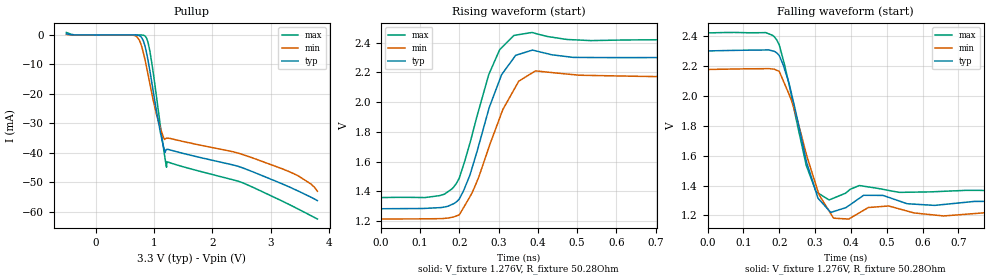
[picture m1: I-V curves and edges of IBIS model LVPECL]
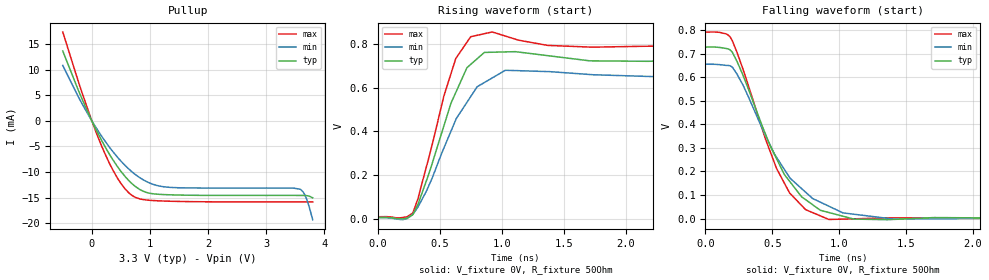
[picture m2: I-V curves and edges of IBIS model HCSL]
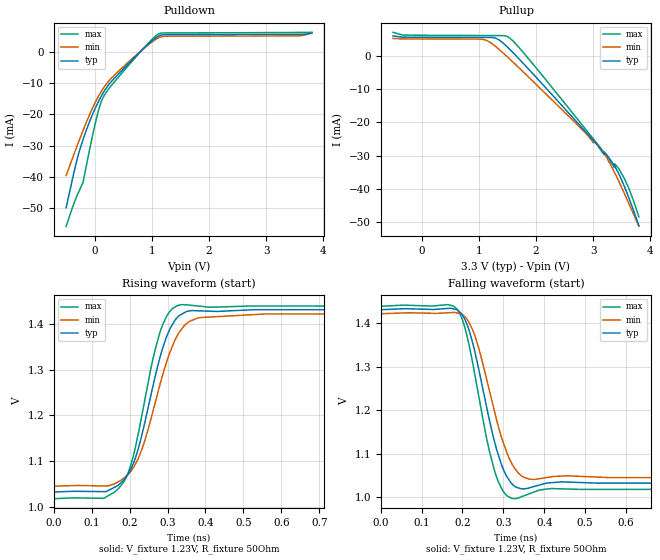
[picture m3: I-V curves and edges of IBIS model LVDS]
|Texas Instruments Incorporated
| Marketing part#   Digital Voltage Range   Package-type   #pins
|   LMK61E2   3.15V - 3.465V
[IBIS Ver]   4.1
[File name]   lmk61e2.ibs
[File Rev]   1.0
[Date]   08/25/2015
[Source]
| Texas Instruments Incorporated.
| 12500 TI Blvd
| Dallas, TX -75243
[Notes]   Revision History:
| Rev 1.0: 08/25/2015
| - Initial version of the model
| - Model generated from simulations in TISPICE
| - C_comp although listed in numerical order of value are
|   obtained from varying PVT conditions. For PVT conditions for
|   each specific value refer the buffer description under
|   respective [Model]. IBIS model user is responsible for using
|   appropriate C_comp to simulate for Signal Integrity.
| - Warnings regarding combined Non-monotonicity of various models have been
|   reviewd and considered minor and can be ignored.
| - Model DRV has sub modles, LVPECL, HCSL, LVDS, depending on the
|   driver mode. User should be able to select a desired driver under
|   [Model Selector].
[Disclaimer]
| This model is designed as an aid for customers of Texas Instruments.
| TI and its licensors and suppliers make no warranties, either expressed
| or implied, with respect to this  model, including the warranties of
| merchantability or fitness for a particular purpose. The model is
| provided solely on an "as is" basis. The entire risk as to its quality
| and performance is with the customer.
[Copyright]
 (C) Copyright 2015 Texas Instruments Incorporated.All rights reserved.
|   Device
[Component] LMK61E2
[Manufacturer]   TI
[Package]
|   typ   min   max
R_pkg   0   0   0
L_pkg   0   0   0
C_pkg   0   0   0
[Pin]  signal_name model_name   R_pin   L_pin   C_pin
1   OE   NC   0   0   0
2   ADD   NC   0   0   0
3   GND   GND   0   0   0
4   OUTP   DRV  0   0   0
5   OUTN   DRV   0   0   0
6   VCC   POWER   0   0   0
7   SDA   NC   0   0   0
8   SCL   NC   0   0   0
[Diff Pin]  inv_pin  vdiff  tdelay_typ tdelay_min tdelay_max
4   5   NA   NA   NA   NA
|   Model Selectors
[Model Selector]  DRV
LVPECL  driver in lvpecl mode
HCSL  driver in hcsl mode
LVDS  driver in lvds mode
| Models and submodels in the file (3): LVPECL (Open_source), HCSL (Open_source), LVDS (Output)
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|   Model
[Model]   LVPECL
Model_type   Open_source
Polarity   Non-Inverting
Vmeas = 1.6
Vref = 1.276
Cref = 1pF
Rref = 50
|   typ   min   max
C_comp   0.215pF   0.202pF   0.225pF
[Voltage Range]   3.3   3.135   3.465
[Temperature Range]   27   85   -40
[Pullup Reference]   3.3   3.135   3.465
[Pulldown Reference]   0   0   0
[Power Clamp Reference]   3.3   3.135   3.465
[GND Clamp Reference]   0   0   0
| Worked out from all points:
|   falling waveform, V_fixture 1.276V, R_fixture 50.28Ohm: 20-80 % time 59.3ps typ, 70.2ps min, 57.1ps max; typ from 2.3 V to 1.29 V
|   rising waveform, V_fixture 1.276V, R_fixture 50.28Ohm: 20-80 % time 72.3ps typ, 83.7ps min, 68.7ps max; typ from 1.28 V to 2.31 V
[Pullup]
|   Voltage   I(typ)   I(min)   I(max)
-500mV    388.3uA    158.6uA    847.9uA
656.7mV   -6.836uA   -136.4uA   -40.3nA
759.9mV   -323uA     -2.236mA   -5.545uA
863.1mV   -5.164mA   -9.896mA   -731.8uA
936.2mV   -12.86mA   -17.1mA    -6.174mA
1.117V    -33.67mA   -32.01mA   -31.83mA
1.19V     -39.75mA   -35.29mA   -41.82mA
1.216V    -38.82mA   -35mA      -44.83mA
1.233V    -38.78mA   -34.98mA   -43.02mA
2.446V    -44.54mA   -40.07mA   -49.58mA
3.465V    -52.84mA   -47.68mA   -58.94mA
3.8V      -56.16mA   -52.97mA   -62.4mA
[Ramp]
R_load = 50.28
|   typ   min   max
dV/dt_r   0.613874/7.22802e-11   0.581205/8.37044e-11   0.635139/6.87025e-11
dV/dt_f   0.605179/9.77e-11   0.573672/7.01775e-11   0.633996/5.71456e-11
[Falling Waveform]
V_fixture = 1.276V
V_fixture_min = 1.212V
V_fixture_max = 1.34V
R_fixture = 50.28Ohm
C_fixture = 0F
|   Time   V(typ)   V(min)   V(max)
0s        2.298V     2.174V     2.418V
162.1ps   2.304V     2.179V     2.42V
200ps     2.267V     2.162V     2.338V
227.2ps   2.083V     2.009V     2.076V
275ps     1.569V     1.615V     1.537V
307.8ps   1.316V     1.362V     1.35V
339.1ps   1.233V     1.23V      1.304V
435.5ps   1.335V     1.235V     1.395V
633.7ps   1.267V     1.203V     1.359V
2ns       1.289V     1.218V     1.361V
[Rising Waveform]
V_fixture = 1.276V
V_fixture_min = 1.212V
V_fixture_max = 1.34V
R_fixture = 50.28Ohm
C_fixture = 0F
|   Time   V(typ)   V(min)   V(max)
0s        1.284V     1.215V     1.359V
149.5ps   1.291V     1.218V     1.372V
200ps     1.349V     1.243V     1.49V
227.2ps   1.511V     1.365V     1.725V
275ps     1.952V     1.694V     2.184V
307.8ps   2.185V     1.929V     2.365V
339.1ps   2.298V     2.083V     2.448V
393.9ps   2.345V     2.21V      2.461V
534.8ps   2.299V     2.179V     2.413V
2ns       2.307V     2.184V     2.418V
|   Model
[Model]   HCSL
Model_type   Open_source
Polarity   Non-Inverting
Vmeas = 0.35
Vref = 0
Cref = 1pF
Rref = 50
|   typ   min   max
C_comp   0.215pF   0.202pF   0.225pF
[Voltage Range]   3.3   3.135   3.465
[Temperature Range]   27   85   -40
[Pullup Reference]   3.3   3.135   3.465
[Pulldown Reference]   0   0   0
[Power Clamp Reference]   3.3   3.135   3.465
[GND Clamp Reference]   0   0   0
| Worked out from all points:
|   slope of the pullup table from 0 to 0.495 V, typ, clamps not added: 50.6 ohm
|   falling waveform, V_fixture 0V, R_fixture 50Ohm: 20-80 % time 347ps typ, 395ps min, 301ps max; typ from 0.728 V to 0 V
|   rising waveform, V_fixture 0V, R_fixture 50Ohm: 20-80 % time 256ps typ, 312ps min, 216ps max; typ from 0.005 V to 0.727 V
[Pullup]
|   Voltage   I(typ)   I(min)   I(max)
-500mV    13.64mA    10.81mA    17.35mA
-164.6mV  4.159mA    3.265mA    5.36mA
11.7mV    -280.2uA   -219.3uA   -362.8uA
175.1mV   -3.963mA   -3.111mA   -5.088mA
441.7mV   -8.953mA   -7.106mA   -11.2mA
575mV     -10.91mA   -8.74mA    -13.33mA
695.4mV   -12.31mA   -9.994mA   -14.59mA
936.2mV   -13.96mA   -11.83mA   -15.45mA
1.297V    -14.42mA   -12.95mA   -15.68mA
3.585V    -14.56mA   -13.35mA   -15.82mA
3.684V    -14.59mA   -14.95mA   -15.82mA
3.8V      -15.04mA   -19.3mA    -15.83mA
[Ramp]
R_load = 50
|   typ   min   max
dV/dt_r   0.433319/2.55754e-10   0.391319/3.11773e-10   0.469787/2.15724e-10
dV/dt_f   0.436287/3.47027e-10   0.392611/3.95051e-10   0.474509/3.01064e-10
[Falling Waveform]
V_fixture = 0V
V_fixture_min = 0V
V_fixture_max = 0V
R_fixture = 50Ohm
C_fixture = 0F
|   Time   V(typ)   V(min)   V(max)
0s        727.5mV    654.7mV    791mV
153.1ps   721.5mV    649.7mV    783.5mV
200ps     706.1mV    642.8mV    755.2mV
448.3ps   358.2mV    352.6mV    337.4mV
531.4ps   253.6mV    259.3mV    212mV
628.2ps   158.4mV    174.6mV    108.8mV
718.1ps   92.33mV    127.1mV    55.52mV
922.3ps   25.37mV    52.16mV    -4.102mV
1.385ns   -4.344mV   -980.1uV   2.966mV
4ns       397.9uV    332.1uV    132.8uV
[Rising Waveform]
V_fixture = 0V
V_fixture_min = 0V
V_fixture_max = 0V
R_fixture = 50Ohm
C_fixture = 0F
|   Time   V(typ)   V(min)   V(max)
0s        5.072mV    4.307mV    8.373mV
282.1ps   18.8mV     19.31mV    25.55mV
398.2ps   184.6mV    134.6mV    252.3mV
531.4ps   423.5mV    322.4mV    560.5mV
628.2ps   578.1mV    453mV      734mV
748.4ps   706.9mV    559.2mV    833.9mV
858.5ps   761.8mV    623.7mV    847.7mV
1.028ns   764.2mV    680mV      836.9mV
1.728ns   723.2mV    659.8mV    785.9mV
4ns       727.3mV    656.5mV    791.4mV
|   Model
[Model]   LVDS
Model_type   Output
Polarity   Non-Inverting
Vmeas = 1.2
Vref = 1.2
Cref = 1pF
Rref = 50
|   typ   min   max
C_comp   0.215pF   0.202pF   0.225pF
[Voltage Range]   3.3   3.135   3.465
[Temperature Range]   27   85   -40
[Pullup Reference]   3.3   3.135   3.465
[Pulldown Reference]   0   -0   -0
[Power Clamp Reference]   3.3   3.135   3.465
[GND Clamp Reference]   0   0   0
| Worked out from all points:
|   slope of the pulldown table from 0 to 0.495 V, typ, clamps not added: 38.6 ohm
|   slope of the pullup table from 0 to 0.495 V, typ, clamps not added: 23.9 kohm
|   falling waveform, V_fixture 1.23V, R_fixture 50Ohm: 20-80 % time 56.9ps typ, 63.1ps min, 51.7ps max; typ from 1.43 V to 1.03 V
|   rising waveform, V_fixture 1.23V, R_fixture 50Ohm: 20-80 % time 71.6ps typ, 80.6ps min, 64.1ps max; typ from 1.03 V to 1.43 V
[Pulldown]
|   Voltage   I(typ)   I(min)   I(max)
-500mV    -49.82mA   -39.53mA   -55.73mA
-306.5mV  -34.24mA   -30mA      -45.81mA
-207.6mV  -28.25mA   -25.31mA   -41.81mA
11.7mV    -17.94mA   -16.09mA   -22.72mA
71.9mV    -15.66mA   -14.02mA   -18.32mA
145mV     -13.21mA   -11.82mA   -14.67mA
269.7mV   -9.983mA   -8.849mA   -11.27mA
575mV     -4.081mA   -3.531mA   -4.699mA
1.078V    4.563mA    4.069mA    5.198mA
1.237V    5.446mA    4.943mA    5.993mA
3.576V    5.556mA    5.083mA    6.146mA
3.8V      5.937mA    6.058mA    6.203mA
[Pullup]
|   Voltage   I(typ)   I(min)   I(max)
-500mV    5.941mA    5.188mA    7.029mA
1.065V    5.497mA    4.921mA    6.056mA
1.297V    5.266mA    2.725mA    6.044mA
1.534V    2.042mA    -893.3uA   5.403mA
3.086V    -27.12mA   -26.94mA   -26.76mA
3.189V    -29.7mA    -29.27mA   -28.99mA
3.241V    -29.8mA    -30.69mA   -30.13mA
3.374V    -33.09mA   -35.05mA   -33.59mA
3.379V    -33.22mA   -35.2mA    -32.49mA
3.473V    -36.36mA   -38.63mA   -34.62mA
3.628V    -42.81mA   -44.51mA   -40.01mA
3.8V      -51.04mA   -51.23mA   -48.41mA
[Ramp]
R_load = 50
|   typ   min   max
dV/dt_r   0.238508/7.12945e-11   0.225343/8.01796e-11   0.252108/6.37996e-11
dV/dt_f   0.237987/5.68532e-11   0.224972/6.277e-11   0.251474/5.1684e-11
[Falling Waveform]
V_fixture = 1.23V
V_fixture_min = 1.23V
V_fixture_max = 1.23V
R_fixture = 50Ohm
C_fixture = 0F
|   Time   V(typ)   V(min)   V(max)
0s        1.43V      1.421V     1.438V
188.6ps   1.429V     1.422V     1.43V
205.9ps   1.408V     1.414V     1.389V
227.5ps   1.345V     1.378V     1.296V
259.8ps   1.204V     1.268V     1.132V
277.2ps   1.132V     1.202V     1.065V
298.1ps   1.069V     1.13V      1.016V
320.6ps   1.032V     1.078V     997.8mV
370.9ps   1.024V     1.041V     1.011V
2ns       1.034V     1.046V     1.019V
[Rising Waveform]
V_fixture = 1.23V
V_fixture_min = 1.23V
V_fixture_max = 1.23V
R_fixture = 50Ohm
C_fixture = 0F
|   Time   V(typ)   V(min)   V(max)
0s        1.033V     1.045V     1.018V
131.5ps   1.034V     1.046V     1.019V
182.9ps   1.058V     1.062V     1.053V
218.3ps   1.115V     1.099V     1.142V
277.2ps   1.318V     1.259V     1.374V
298.1ps   1.373V     1.319V     1.418V
326.7ps   1.415V     1.376V     1.44V
378.8ps   1.429V     1.413V     1.439V
560.6ps   1.431V     1.422V     1.439V
2ns       1.43V      1.421V     1.438V
